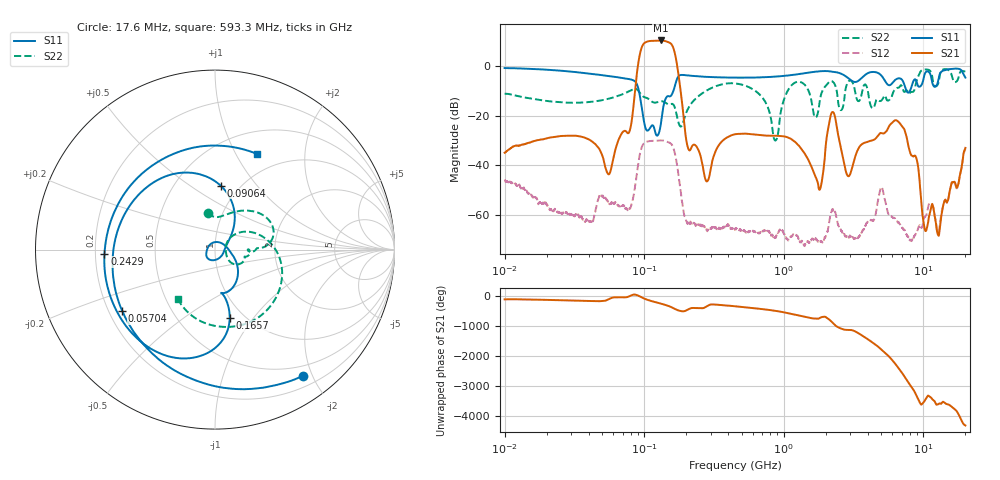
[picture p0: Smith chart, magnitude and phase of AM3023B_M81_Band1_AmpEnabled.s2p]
!Agilent Technologies,E8364B,MY43040894,A.07.50.67
!Agilent E8364B: A.07.50.67
!Date: Tuesday, October 27, 2020 10:42:41
!Correction: S11(Full 2 Port(1,2))
!S21(Full 2 Port(1,2))
!S12(Full 2 Port(1,2))
!S22(Full 2 Port(1,2))
!S2P File: Measurements: S11, S21, S12, S22:Log Frequency Sweep
# Hz S  dB  R 50
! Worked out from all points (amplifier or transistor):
!   3201 points, 10 MHz to 20 GHz, reference 50 ohm
!   highest |S21| = 10.3 dB at 131.3 MHz (marker M1)
!   |S21| within 3 dB of that: 95.72 MHz to 161.7 MHz (65.96 MHz wide, 51.3 % of centre)
!   unconditionally stable (mu >= 1): start of sweep to end of sweep
!   at 35.47 MHz: K = 6575.63, MAG = -25.0 dB, |S12| = -60.8 dB
!   at 447.2 MHz: K = 12141.14, MAG = -24.8 dB, |S12| = -65.7 dB
!   at 20 GHz: K = 291.81, MAG = -27.4 dB, |S12| = -33.5 dB
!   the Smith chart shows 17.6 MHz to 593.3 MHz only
!   S11 on the Smith chart (normalised r, x): 17.6 MHz: 0.35, -1.87; 57.04 MHz: 0.25, -0.28; 90.64 MHz: 0.82, +0.67; 165.7 MHz: 0.86, -0.77; 242.9 MHz: 0.24, -0.02; 593.3 MHz: 0.76, +1.22
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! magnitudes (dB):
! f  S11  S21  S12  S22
! 10 MHz  -0.9  -35.0  -46.0  -11.2
! 17.6 MHz  -1.3  -29.8  -55.3  -13.7
! 35.55 MHz  -2.7  -28.5  -60.9  -14.8
! 57.04 MHz  -4.2  -42.8  -55.6  -13.1
! 90.64 MHz  -8.9  1.0  -39.4  -10.0
! 126.1 MHz  -27.6  10.2  -30.1  -14.5
! 131.3 MHz  -23.8  10.3  -30.0  -14.2
! 165.7 MHz  -8.2  5.2  -35.1  -16.8
! 204.2 MHz  -3.8  -32.3  -63.6  -17.7
! 242.9 MHz  -4.2  -33.5  -64.0  -12.3
! 447.2 MHz  -4.7  -27.5  -65.7  -7.0
! 593.3 MHz  -4.7  -27.6  -66.9  -9.2
! 869.7 MHz  -4.3  -28.1  -69.1  -30.0
! 1.151 GHz  -3.6  -29.8  -68.2  -7.5
! 1.59 GHz  -2.5  -41.0  -69.6  -15.1
! 1.838 GHz  -2.1  -48.8  -70.6  -12.1
! 2.228 GHz  -2.3  -18.6  -57.7  -6.2
! 2.9 GHz  -4.9  -44.4  -68.9  -6.3
! 5.639 GHz  -7.7  -24.5  -59.8  -13.9
! 8.876 GHz  -5.9  -36.9  -67.2  -6.6
! 10.41 GHz  -2.5  -66.5  -60.3  -1.4
! 20 GHz  -4.7  -33.0  -33.5  -2.3
